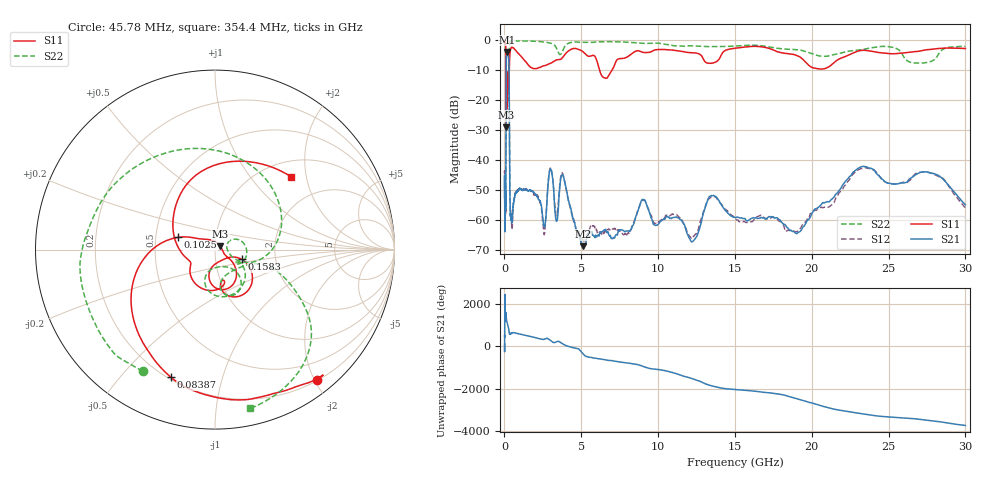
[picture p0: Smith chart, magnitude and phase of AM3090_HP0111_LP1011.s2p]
! Date/Time: Thu, Feb 28, 2019 2:01 PM
! Network Analyzer: Agilent Technologies E8364B Rev: A.07.50.67
! Sweep from 0.010 to 30.000 GHz, 1601 Points, Sweep Type: LOG
! Power Supply: 5.023 V, 0.002 A
# Hz S DB R 50
!freq MagS11 AngS11 MagS21 AngS21 MagS12 AngS12 MagS22 AngS22
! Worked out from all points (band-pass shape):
!   1601 points, 10 MHz to 30 GHz, reference 50 ohm
!   highest |S21| = -4.00 dB at 163.2 MHz (marker M1); lowest = -68.7 dB at 5.103 GHz (marker M2)
!   |S21| within 3 dB of the highest: 114.7 MHz to 285.6 MHz (170.9 MHz wide, 85.4 % of centre)
!   lowest |S11| = -29.1 dB at 110.4 MHz (marker M3), VSWR 1.07, Z = 53.1 + j1.88 ohm
!   |S11| at or under -10 dB: 100.6 MHz to 314.3 MHz (213.7 MHz wide, 103 % of centre); 6.184 GHz to 7.009 GHz (825.1 MHz wide, 12.5 % of centre)
!   |S22| runs from -23.5 to -0.2 dB; largest |S21 - S12| = 0.011
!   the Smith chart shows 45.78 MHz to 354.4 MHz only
!   S11 on the Smith chart (normalised r, x): 45.78 MHz: 0.21, -2.03; 83.87 MHz: 0.21, -0.69; 102.5 MHz: 0.65, +0.09; 158.3 MHz: 1.34, -0.15; 354.4 MHz: 1.32, +1.64
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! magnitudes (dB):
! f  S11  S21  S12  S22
! 10 MHz  -0.2  -46.4  -44.7  -0.7
! 38.04 MHz  -0.5  -60.4  -59.0  -1.6
! 45.78 MHz  -0.7  -55.3  -54.1  -2.1
! 83.87 MHz  -2.5  -53.1  -51.8  -4.7
! 102.5 MHz  -13.2  -16.4  -16.5  -12.4
! 110.4 MHz  -29.1  -8.5  -8.5  -23.3
! 144.7 MHz  -22.6  -4.4  -4.3  -17.1
! 158.3 MHz  -16.0  -4.0  -4.0  -15.8
! 163.2 MHz  -13.6  -4.0  -4.0  -14.5
! 290.1 MHz  -15.3  -7.7  -7.7  -15.1
! 354.4 MHz  -4.6  -51.9  -52.1  -0.9
! 550.5 MHz  -2.6  -55.8  -57.1  -0.3
! 2.084 GHz  -9.6  -51.6  -51.3  -0.5
! 2.571 GHz  -8.6  -61.9  -64.1  -0.7
! 2.958 GHz  -7.8  -43.3  -43.0  -1.0
! 3.385 GHz  -6.6  -60.4  -58.5  -2.7
! 3.798 GHz  -5.8  -45.0  -44.7  -3.5
! 5.103 GHz  -3.9  -68.7  -66.4  -0.8
! 7.926 GHz  -5.8  -63.7  -64.8  -0.7
! 18.93 GHz  -5.0  -64.3  -63.9  -3.2
! 23.48 GHz  -3.4  -42.2  -42.5  -3.0
! 30 GHz  -2.8  -54.9  -55.9  -2.1
